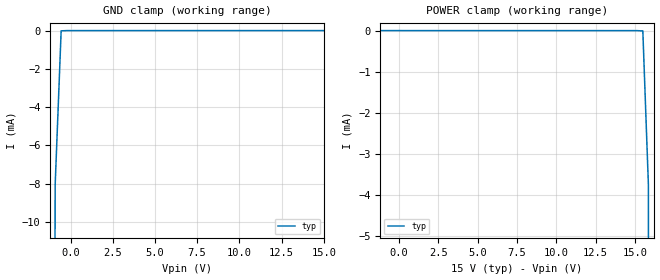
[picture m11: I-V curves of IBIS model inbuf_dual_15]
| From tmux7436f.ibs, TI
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| inbuf_dual_15
[Model]   inbuf_dual_15
Model_type   Input
Vinl = 0.8
Vinh = 1.3
|   typ   min   max
C_comp   6.362683e-13   NA   NA
[Voltage Range]   15   NA   NA
[Temperature Range]   27   NA   NA
[Power Clamp Reference]   15   NA   NA
[GND Clamp Reference]   0   NA   NA
[GND Clamp]
|   Voltage   I(typ)   I(min)   I(max)
-20V      -9.607A    NA         NA
-1.263V   -115.5mA   NA         NA
-909.1mV  -8.044mA   NA         NA
-555.6mV  -13.27uA   NA         NA
15V       1.075uA    NA         NA
[POWER Clamp]
|   Voltage   I(typ)   I(min)   I(max)
-5V       1.354uA    NA         NA
15.51V    -7.864uA   NA         NA
15.86V    -3.749mA   NA         NA
16.21V    -94.01mA   NA         NA
30V       -7.065A    NA         NA
